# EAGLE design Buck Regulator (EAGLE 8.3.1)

## Sheet 1 of 2: DataSheet
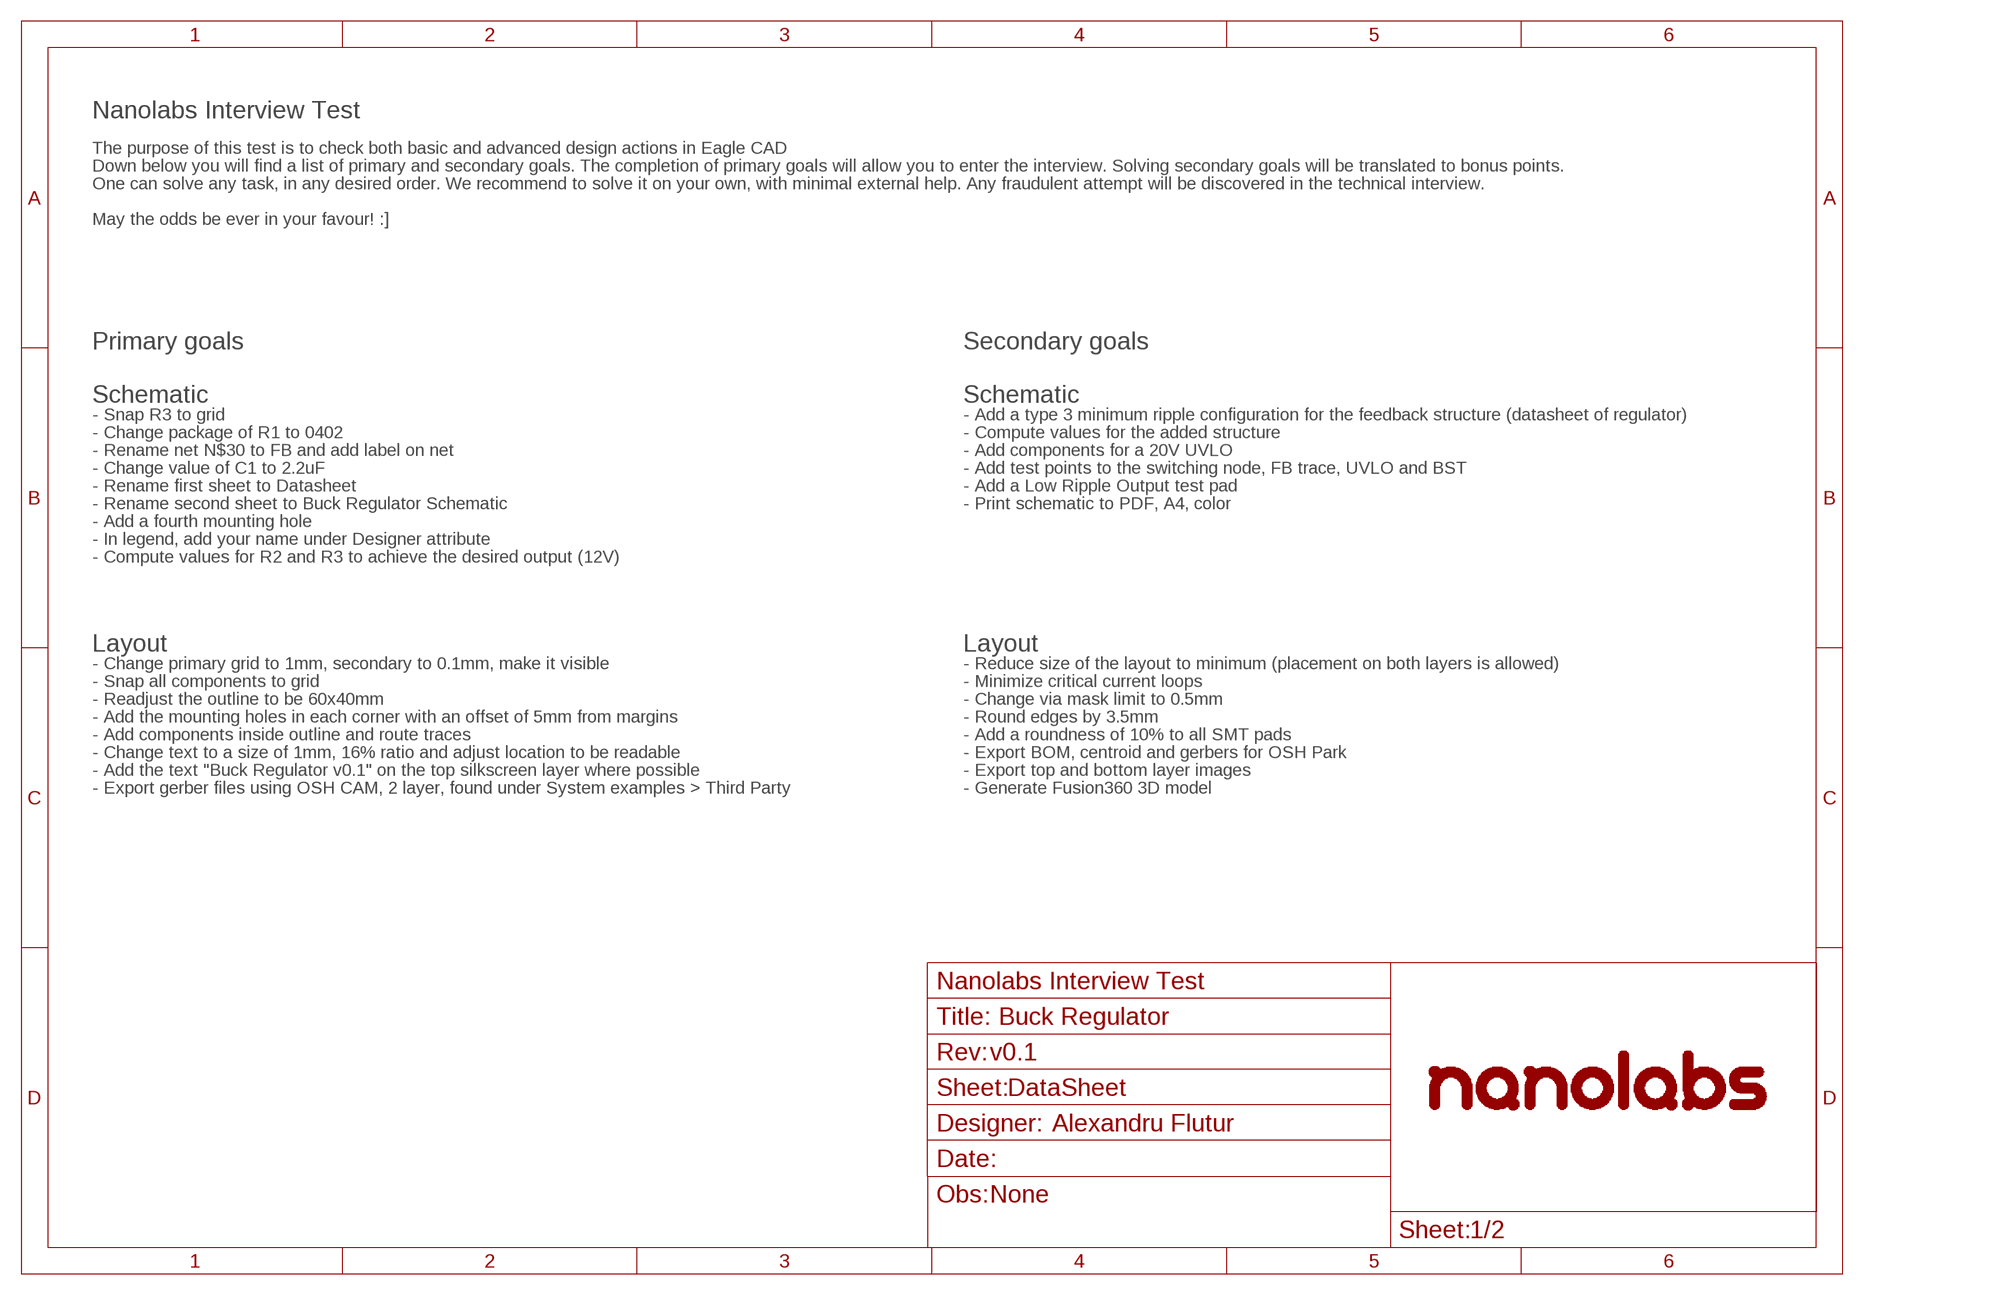
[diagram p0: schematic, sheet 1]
FRAME3 (_SCH_FRAME_A4): OBS: None; REVNUM: v0.1

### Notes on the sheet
- Nanolabs Interview Test
- The purpose of this test is to check both basic and advanced design actions in Eagle CAD
- Down below you will find a list of primary and secondary goals. The completion of primary goals will allow you to enter the interview. Solving secondary goals will be translated to bonus points.
- One can solve any task, in any desired order. We recommend to solve it on your own, with minimal external help. Any fraudulent attempt will be discovered in the technical interview.
- May the odds be ever in your favour! :]
- Primary goals | Secondary goals
- Schematic | Schematic
- - Snap R3 to grid | - Add a type 3 minimum ripple configuration for the feedback structure (datasheet of regulator)
- - Change package of R1 to 0402 | - Compute values for the added structure
- - Rename net N$30 to FB and add label on net | - Add components for a 20V UVLO
- - Change value of C1 to 2.2uF | - Add test points to the switching node, FB trace, UVLO and BST
- - Rename first sheet to Datasheet | - Add a Low Ripple Output test pad
- - Rename second sheet to Buck Regulator Schematic | - Print schematic to PDF, A4, color
- - Add a fourth mounting hole
- - In legend, add your name under Designer attribute
- - Compute values for R2 and R3 to achieve the desired output (12V)
- Layout | Layout
- - Change primary grid to 1mm, secondary to 0.1mm, make it visible | - Reduce size of the layout to minimum (placement on both layers is allowed)
- - Snap all components to grid | - Minimize critical current loops
- - Readjust the outline to be 60x40mm | - Change via mask limit to 0.5mm
- - Add the mounting holes in each corner with an offset of 5mm from margins | - Round edges by 3.5mm
- - Add components inside outline and route traces | - Add a roundness of 10% to all SMT pads
- - Change text to a size of 1mm, 16% ratio and adjust location to be readable | - Export BOM, centroid and gerbers for OSH Park
- - Add the text "Buck Regulator v0.1" on the top silkscreen layer where possible | - Export top and bottom layer images
- - Export gerber files using OSH CAM, 2 layer, found under System examples > Third Party | - Generate Fusion360 3D model
- Alexandru Flutur

## Sheet 2 of 2: Buck Regulator Schematic
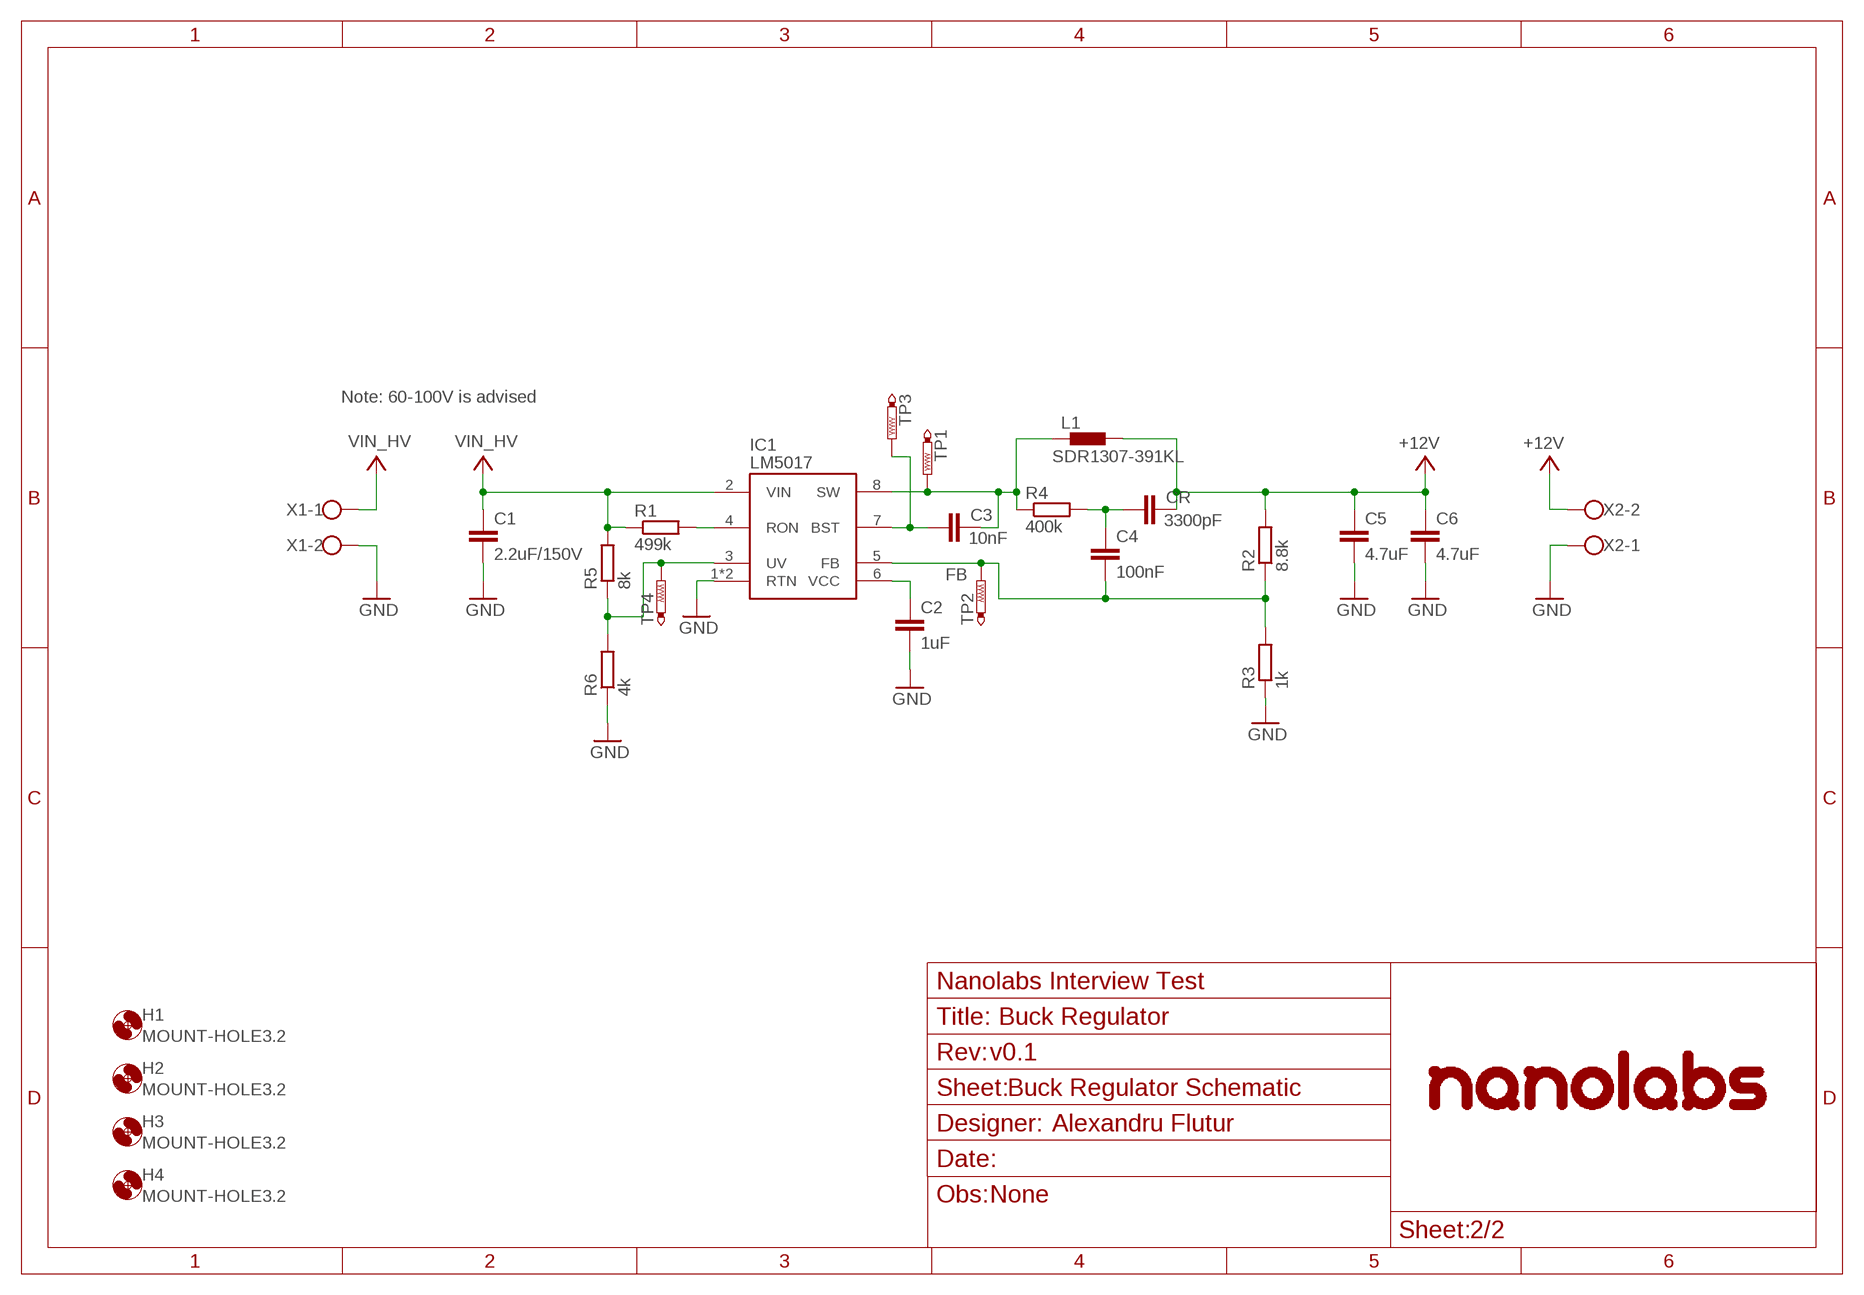
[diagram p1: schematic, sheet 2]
FRAME1 (_SCH_FRAME_A4): OBS: None; REVNUM: v0.1

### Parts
C1  2.2uF/150V  C-EUC1812  [C1812]
C2  1uF  C-EUC0603  [C0603]
C3  10nF  C-EUC0603  [C0603]
C4  100nF  C-EUC0603  [C0603]
C5  4.7uF  C-EUC0603  [C0603]
C6  4.7uF  C-EUC0603  [C0603]
CR  3300pF  C-EUC0603  [C0603]
H1  MOUNT-HOLE3.2  [3,2]
H2  MOUNT-HOLE3.2  [3,2]
H3  MOUNT-HOLE3.2  [3,2]
H4  MOUNT-HOLE3.2  [3,2]
IC1  LM5017  [SO-08-EP]
L1  SDR1307-391KL  [SDR1307-391KL]
R1  499k  R-EU_R0402  [R0402]
R2  8.8k  R-EU_R0603  [R0603]
R3  1k  R-EU_R0603  [R0603]
R4  400k  R-EU_R0402  [R0402]
R5  8k  R-EU_R0603  [R0603]
R6  4k  R-EU_R0603  [R0603]
TP1  PTR1B1,27  [B1,27]
TP2  PTR1B1,27  [B1,27]
TP3  PTR1B1,27  [B1,27]
TP4  PTR1B1,27  [B1,27]
X1  W237-102  [W237-102]
X2  W237-102  [W237-102]

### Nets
+12V: C5.1 C6.1 CR.2 L1.2 R2.2 X2.2
FB: C4.2 IC1.5(FB) R2.1 R3.2 TP2.TP
GND: C1.2 C2.2 C5.2 C6.2 IC1.1(RTN) IC1.9(RTN) R3.1 R6.1 X1.2 X2.1
N$1: C4.1 CR.1 R4.2
N$2: IC1.3(UV) R5.1 R6.2 TP4.TP
N$23: C2.1 IC1.6(VCC)
N$28: C3.1 IC1.7(BST) TP3.TP
N$29: C3.2 IC1.8(SW) L1.1 R4.1 TP1.TP
N$31: IC1.4(RON) R1.2
VIN_HV: C1.1 IC1.2(VIN) R1.1 R5.2 X1.1

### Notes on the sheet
- Note: 60-100V is advised
- Alexandru Flutur

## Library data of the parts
C1-C6 CR = rcl:C-EU: CAPACITOR, European symbol; SPICEPREFIX: C
H1-H4 = _nanolabs_layout:MOUNT-HOLE: MOUNTING HOLE with drill center marker
IC1 = _nanolabs_ic:LM5017
L1 = _nanolabs_rcl:SDR1307-391KL
R1-R6 = rcl:R-EU_: RESISTOR, European symbol; SPICEPREFIX: R
TP1-TP4 = testpad:PTR1: TEST PIN
X1 X2 = con-wago-500:W237-102: WAGO SCREW CLAMP; MPN: 237-102; OC_FARNELL: unknown; OC_NEWARK: 70K9898

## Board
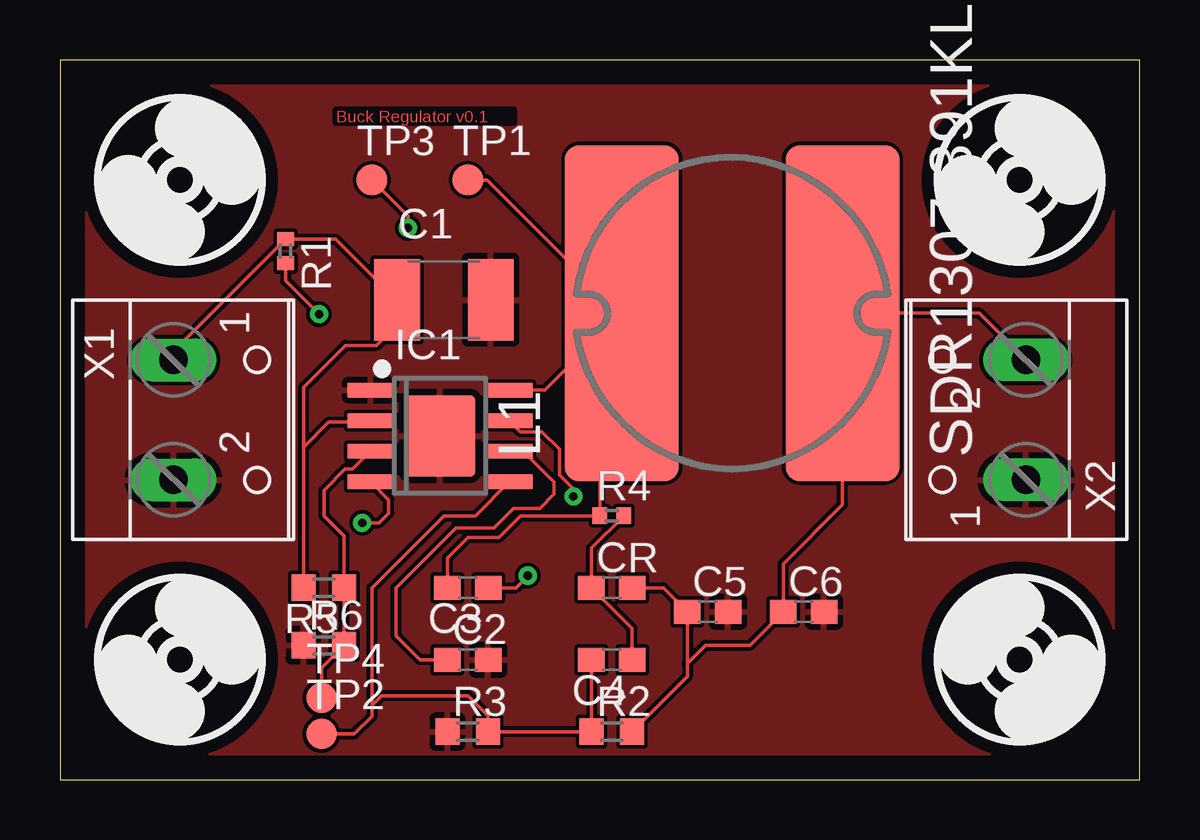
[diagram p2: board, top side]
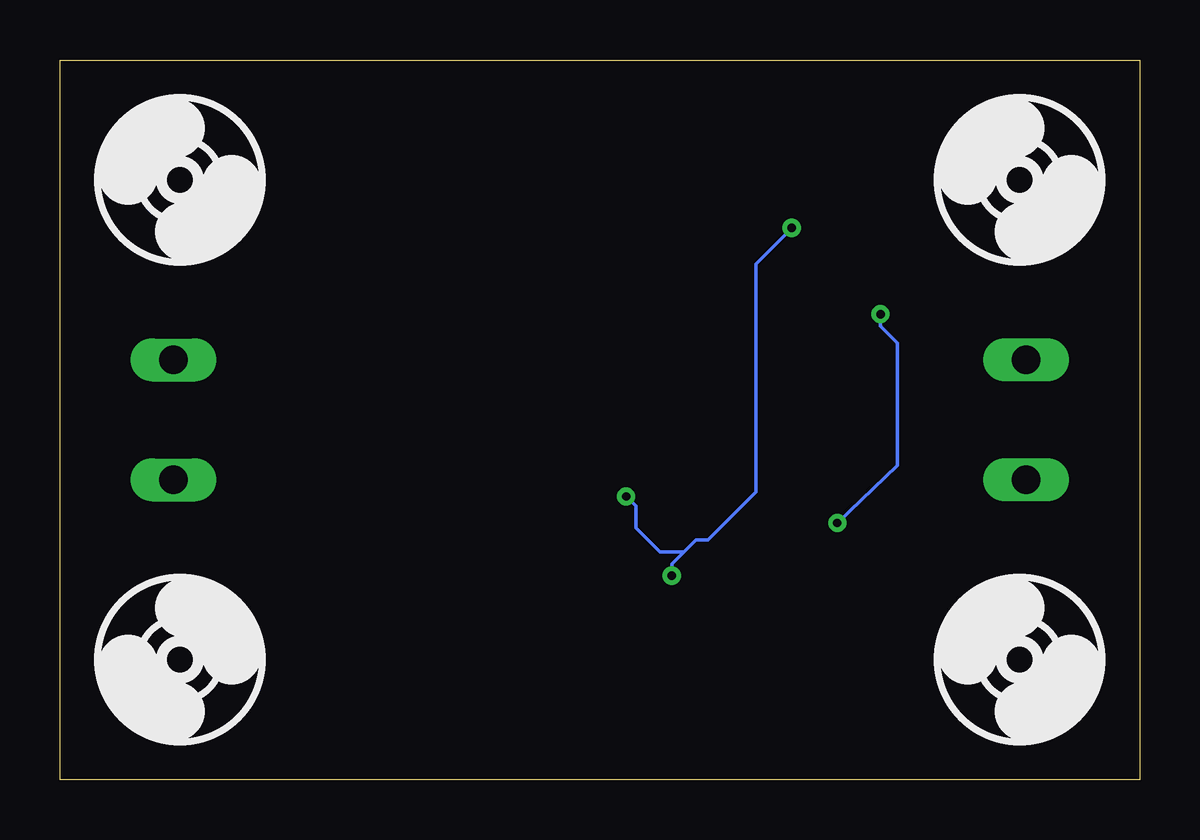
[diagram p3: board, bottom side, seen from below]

Size 45 x 30 mm. Coordinates in mm from the lower left corner, seen from the top.
Outline: 0,0 45,0 45,30 0,30 0,0
Copper layers (1*16): Top 0.035mm / dielectric 1.5mm / Bottom 0.035mm
Design rules "default": minimum track width 6mil, minimum drill 0.35mm, track to track 6mil, track to pad 6mil, pad to pad 6mil, via to via 6mil, smd to smd 6mil, copper to edge 40mil, drill to drill 6mil, minimum pad ring 10mil, minimum via ring 8mil, stop-mask expansion 4mil, vias tented up to drill 0mil, thermal gap 10mil

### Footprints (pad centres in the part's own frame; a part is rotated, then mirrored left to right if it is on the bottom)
C1812 = smd 1.9 x 3.4: 1 -1.95,0; 2 1.95,0
C0603 = smd 1.1 x 1: 1 -0.85,0; 2 0.85,0
3,2 = hole 3.2: 0,0
SO-08-EP = smd 0.6 x 1.9: 1 -1.905,-2.9; 2 -0.635,-2.9; 3 0.635,-2.9; 4 1.905,-2.9; 5 1.905,2.9; 6 0.635,2.9; 7 -0.635,2.9; 8 -1.905,2.9 | smd 3.4 x 2.95: 9 0,0
SDR1307-391KL = smd 14 x 4.75: 1 0,4.6; 2 0,-4.6
R0402 = smd 0.6 x 0.7: 1 -0.5,0; 2 0.5,0
R0603 = smd 1 x 1.1: 1 -0.85,0; 2 0.85,0
B1,27 = smd 1.27 x 1.27: TP 0,0
W237-102 = drill 1.194 long: 1 -2.5,-1.27; 2 2.5,-1.27

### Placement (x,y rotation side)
C1  16,20 0 top
C2  17,5 0 top
C3  17,8 180 top
C4  23,5 180 top
C5  27,7 0 top
C6  31,7 0 top
CR  23,8 0 top
H1  40,5 270 top
H2  40,25 0 top
H3  5,25 0 top
H4  5,5 0 top
IC1  15.84,14.33 270 top
L1  28.02,19.44 90 top
R1  9.4,22.03 270 top
R2  23,2 0 top
R3  17,2 0 top
R4  23,11 0 top
R5  11,8 180 top
R6  11,5.6 0 top
TP1  17,25 0 top
TP2  10.9,1.9 0 top
TP3  13,25 0 top
TP4  10.9,3.4 0 top
X1  6,15 270 top
X2  39,15 90 top

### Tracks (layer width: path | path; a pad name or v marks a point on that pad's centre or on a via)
+12V
  Top 0.152: X2.2 38.33,19.44 L1.2 32.62,11.47 30.15,9 C6.1 28.75,5.6 26.9,5.6 26.15,4.85 26.15,4.8 | 26.15,4.8 C5.1 25.15,8 CR.2 | 26.15,4.8 26.15,4.3 R2.2
FB
  Top 0.152: R3.2 R2.1 C4.2 | 17.85,1.85 R3.2 | IC1.5 17.32,11 16,11 13,8 13,3.1 | 13,3.1 13,2.63 12.27,1.9 TP2.TP | R3.2 17.85,2.65 17,3.5 13.4,3.5 13,3.1
GND
  pour Top: 0.1,30.1 45,30.1 45.1,30 45.1,-0.1 -0.1,-0.1 -0.1,29.9
N$1
  Top 0.152: 23.85,5.3 C4.1 23.85,6.3 CR.1 22.15,9.65 R4.2
N$2
  Top 0.152: IC1.3 12.2,12.95 11.89,12.95 11,12.06 11,11 11.85,10.15 R5.1 R6.2 10.9,4.65 TP4.TP
N$23
  Top 0.152: IC1.6 19.3,13.7 20.6,12.4 20.6,11.9 20,11.3 19.07,11.3 18.9,11.3 18.1,10.5 16.5,10.5 14,8 14,6 15,5 C2.1
N$28  (via drill 0.35)
  Top 0.152: C3.1 19,8 v19.5,8.5 | v14.5,23 14.5,23.5 TP3.TP | v21.4,11.8 21.4,12.11 20.82,12.69 20.82,13.78 20.1,14.5 19.2,14.5 IC1.7
  Bottom 0.152: v19.5,8.5 19.5,9 19,9.5 | 19,9.5 18.5,10 18,10 16,12 16,21.5 v14.5,23 | 19,9.5 20,9.5 21,10.5 21,11.4 v21.4,11.8
N$29
  Top 0.152: IC1.8 20.21,16.23 23.39,19.41 | 23.39,19.41 L1.1 | 23.39,19.41 23.5,19.3 23.5,18 22.5,17 R4.1 19.2,11 18.3,10.1 17,10.1 16.15,9.25 C3.2 | TP1.TP 17.8,25 23.39,19.41
N$31  (via drill 0.35)
  Top 0.152: R1.2 9.4,20.8 v10.8,19.4 | 12.9,12.38 IC1.4 13.7,11.66 13.7,11.1 13.3,10.7 v12.6,10.7
  Bottom 0.152: v10.8,19.4 10.8,18.9 10.1,18.2 10.1,13.1 v12.6,10.7
VIN_HV
  Top 0.152: 14.02,19.97 14.03,19.98 | 14.02,19.97 13.58,19.53 | 14.03,19.98 C1.1 | IC1.2 12.9,15 12.8,14.9 11.2,14.9 10.15,13.85 10.15,13.8 | X1.1 4.73,17.86 R1.1 11.49,22.53 14.03,19.98 | 14.02,19.97 13.5,19.45 13.5,18.4 13.2,18.1 11.9,18.1 10.15,16.35 10.15,13.8 | R5.2 10.15,13.8

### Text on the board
Top: Buck Regulator v0.1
